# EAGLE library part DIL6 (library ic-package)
Dual In Line / Socket
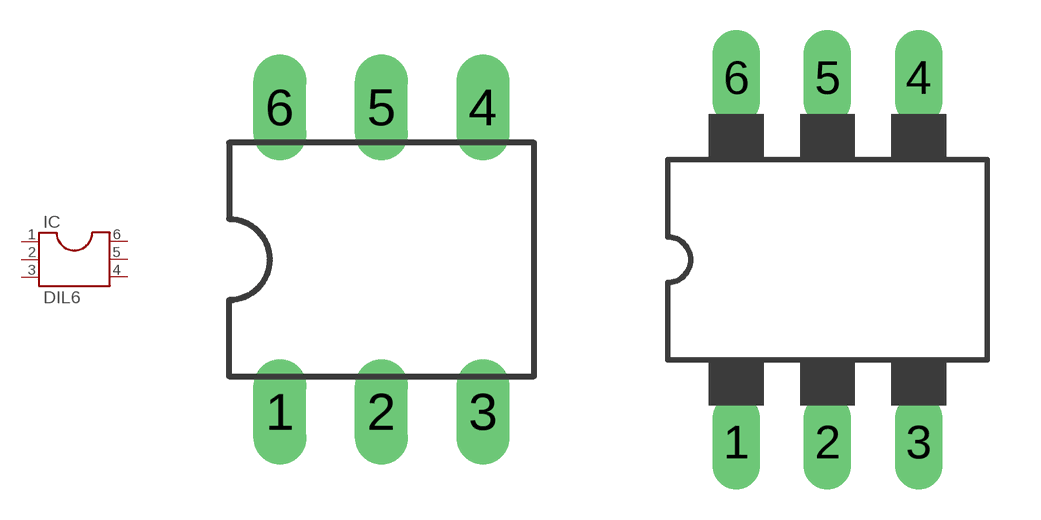
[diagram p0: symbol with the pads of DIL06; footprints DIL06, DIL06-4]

Designator prefix IC

## DIL6  [DIL06]
1  1  pas
2  2  pas
3  3  pas
4  4  pas
5  5  pas
6  6  pas

## DIL6/4  [DIL06-4]
Pads as for DIL06

## DIL6S  [SOCKET-06]
Pads as for DIL06

## Footprint DIL06 (pad centres in mm)
Dual In Line Package
drill 0.813 long: 1 -2.54,-3.81; 2 0,-3.81; 3 2.54,-3.81; 4 2.54,3.81; 5 0,3.81; 6 -2.54,3.81

## Footprint DIL06-4 (pad centres in mm)
Dual In Line Package 0.4 inch
drill 0.813 long: 1 -2.54,-5.08; 2 0,-5.08; 3 2.54,-5.08; 4 2.54,5.08; 5 0,5.08; 6 -2.54,5.08

## Footprint SOCKET-06 (pad centres in mm)
Dual In Line Socket
drill 0.813 long: 1 -2.54,-3.81; 2 0,-3.81; 3 2.54,-3.81; 4 2.54,3.81; 5 0,3.81; 6 -2.54,3.81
